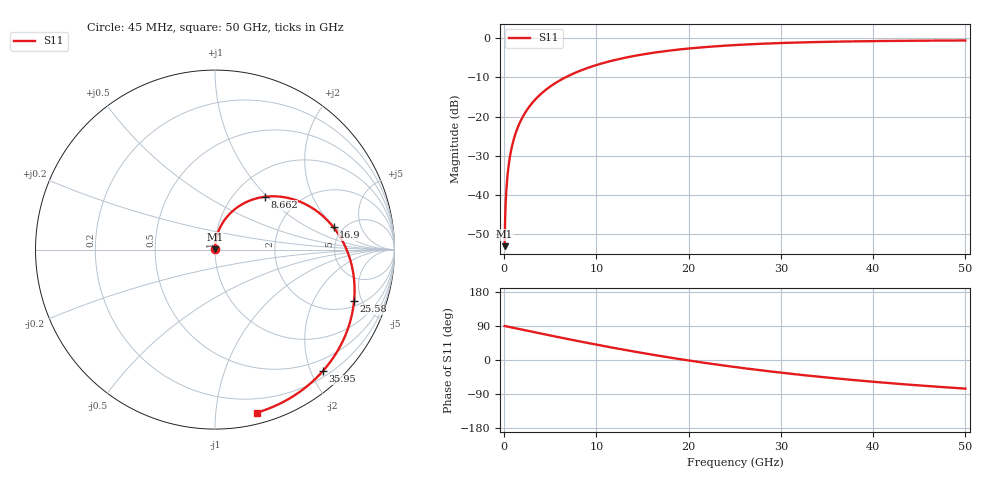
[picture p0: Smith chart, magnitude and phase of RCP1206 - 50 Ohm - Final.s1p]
!Vishay Electro-Films Inc.
!RCP Family
!Case Size 1206
!Assembly Style Surface Mount
!11/2/2015
!efi@vishay.com
# GHz S MA R 50
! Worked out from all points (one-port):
!   801 points, 45 MHz to 50 GHz, reference 50 ohm
!   lowest |S11| = -53.0 dB at 45 MHz (marker M1), VSWR 1.00, Z = 50 + j0.224 ohm
!   |S11| at or under -10 dB: start of sweep to 6.613 GHz
!   S11 on the Smith chart (normalised r, x): 45 MHz: 1.00, +0.00; 8.662 GHz: 1.37, +0.96; 16.9 GHz: 4.20, +1.90; 25.58 GHz: 2.38, -4.31; 35.95 GHz: 0.29, -2.19; 50 GHz: 0.09, -1.29
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0.045  0.002239 89.8
0.1698875  0.008451 89.1
0.3572187  0.01777 88.2
0.4196625  0.02087 87.9
0.54455  0.02708 87.2
0.7318813  0.03639 86.3
0.9192125  0.04569 85.3
1.168988  0.05808 84.0
1.481206  0.07354 82.4
1.855869  0.09203 80.5
2.292975  0.1135 78.3
3.354519  0.1652 72.9
4.665838  0.2275 66.4
6.289375  0.3019 58.3
8.662237  0.4032 46.8
10.53555  0.4761 38.1
12.53375  0.5462 29.0
14.59439  0.6102 20.1
16.90481  0.6721 10.6
18.77812  0.7151 3.3
21.83787  0.773 -7.9
25.0225  0.8192 -18.5
25.58449  0.8261 -20.3
31.26687  0.879 -36.8
35.95016  0.9054 -48.5
37.51125  0.9118 -52.1
43.75563  0.9291 -64.8
50  0.9378 -75.5
